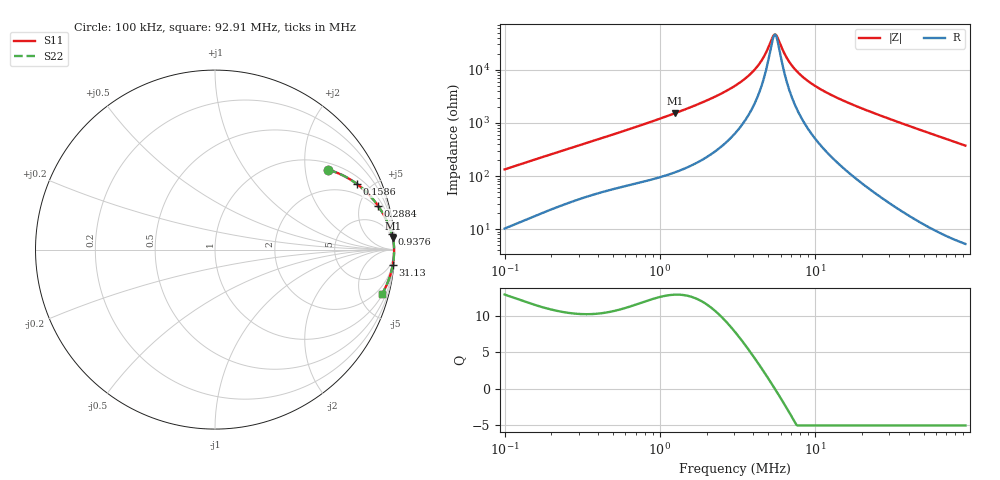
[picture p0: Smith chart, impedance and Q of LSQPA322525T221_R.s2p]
! LSQPA322525T221_R  S-PARAMETER MODEL  ( General Type )
! Model Generated by TAIYO YUDEN Corporation (http://www.ty-top.com)
! Version 1.0
! TAIYO YUDEN Control No. 111018NG25SB-FKC
! Copyright(c) 2011 TAIYO YUDEN CO.,LTD. All Rights Reserved.
! Product Description (link to TY-COMPAS)
! https://ds.yuden.co.jp/TYCOMPAS/or/detail?pn=LSQPA322525T221KR&u=M
! Products Name : Inductors
! Characteristics :
!  Inductance : 220 uH , SRF(min) : 3.0 MHz , DC Resistance(max) : 3.25 Ohm
!  Rated Current : Saturation :190 mA , Temp Rise : 190 mA (40 degC)
!  Case Size : 3.2 x 2.5 / 0.126 x 0.098 [mm/inch] , Thickness : 2.5 / 0.098 [mm/inch]
!  (Conditions: Temperature = 25 degC , DC Bias Current/Voltage = 0A / 0V)
! External Node Assignments :
!  1  o---GGG---o  2
! GND o---------o GND
! Frequency Range : 0.1MHz  -  92.907885MHz  [ 402 STEP ]
# MHz S RI R 50
! Freq[MHz].  S11 Real  S11 Imag  S21 Real  S21 Imag  S12 Real  S12 Imag  S22 Real  S22 Imag
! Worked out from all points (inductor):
!   401 points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, 100 kHz to 92.91 MHz, reference 50 ohm
!   read as one part in series: L = 209 uH near 103.5 kHz
!   highest Q = 12.9 at 1.254 MHz (marker M1), where L = 193 uH
!   self-resonance near 5.449 MHz
!   S11 on the Smith chart (normalised r, x): 100 kHz: 1.21, +2.66; 158.6 kHz: 1.36, +4.13; 288.4 kHz: 1.70, +7.22; 937.6 kHz: 3, +22; 31.13 MHz: 2, -23; 92.91 MHz: 1.11, -7.49
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0.1  0.6312 0.4453  0.3688 -0.4453  0.3688 -0.4453  0.6312 0.4453
0.158615  0.7914 0.3649  0.2086 -0.3649  0.2086 -0.3649  0.7914 0.3649
0.288435  0.9091 0.2429  0.0909 -0.2429  0.0909 -0.2429  0.9091 0.2429
0.314158  0.9196 0.2274  0.0804 -0.2274  0.0804 -0.2274  0.9196 0.2274
0.937642  0.9853 0.0868  0.0147 -0.0868  0.0147 -0.0868  0.9853 0.0868
0.986956  0.9864 0.0825  0.0136 -0.0825  0.0136 -0.0825  0.9864 0.0825
1.253659  0.9908 0.0645  0.00924 -0.0645  0.00924 -0.0645  0.9908 0.0645
2.129137  0.9957 0.0346  0.00431 -0.0346  0.00431 -0.0346  0.9957 0.0346
3.100605  0.9971 0.0192  0.0029 -0.0192  0.0029 -0.0192  0.9971 0.0192
4.21705  0.9976 0.00856  0.00236 -0.00856  0.00236 -0.00856  0.9976 0.00856
4.672288  0.9977 0.00525  0.00226 -0.00525  0.00226 -0.00525  0.9977 0.00525
5.356617  0.9978 0.000902  0.00217 -0.000902  0.00217 -0.000902  0.9978 0.000902
5.542821  0.9978 -0.000179  0.00216 0.000179  0.00216 0.000179  0.9978 -0.000179
5.735498  0.9978 -0.00126  0.00215 0.00126  0.00215 0.00126  0.9978 -0.00126
6.354654  0.9979 -0.00452  0.00214 0.00452  0.00214 0.00452  0.9979 -0.00452
7.04065  0.9978 -0.00782  0.00216 0.00782  0.00216 0.00782  0.9978 -0.00782
8.071863  0.9978 -0.0124  0.00223 0.0124  0.00223 0.0124  0.9978 -0.0124
9.575801  0.9976 -0.0184  0.0024 0.0184  0.0024 0.0184  0.9976 -0.0184
14.93133  0.9966 -0.037  0.00343 0.037  0.00343 0.037  0.9966 -0.037
30.08319  0.9909 -0.0829  0.00911 0.0829  0.00911 0.0829  0.9909 -0.0829
31.12893  0.9904 -0.0859  0.00964 0.0859  0.00964 0.0859  0.9904 -0.0859
92.90788  0.9304 -0.2475  0.0696 0.2475  0.0696 0.2475  0.9304 -0.2475
